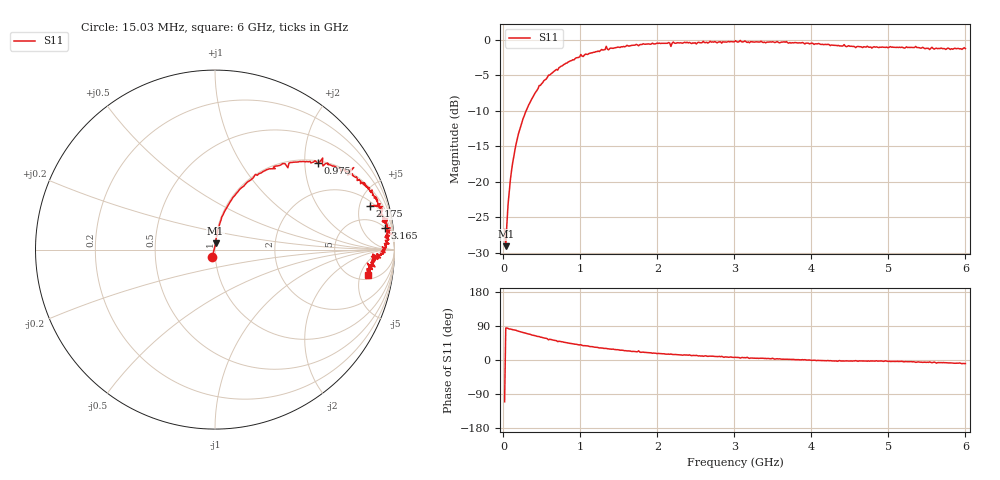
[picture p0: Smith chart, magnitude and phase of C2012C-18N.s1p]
!	Network	Analyzer	HP8753E.07.74:	Oct	30	2002	Serial	No.	JP38451487
!	Hewlett-Packard
!	7	Sep	2009	10:46:32
!	Frequency	S11
#	HZ	S	RI	R	50
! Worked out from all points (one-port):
!   400 points, 15.03 MHz to 6 GHz, reference 50 ohm
!   lowest |S11| = -29.1 dB at 30.03 MHz (marker M1), VSWR 1.07, Z = 50.2 + j3.51 ohm
!   |S11| at or under -10 dB: start of sweep to 295.5 MHz
!   S11 on the Smith chart (normalised r, x): 15.03 MHz: 0.97, -0.08; 975 MHz: 1.06, +2.33; 2.175 GHz: 2.52, +6.25; 3.165 GHz: 5, +14; 6 GHz: 6.09, -6.85
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1.502992e7  -0.0159 -0.0431
3.002985e7  0.00348 0.0349
6.00297e7  0.00803 0.0687
1.050295e8  0.0191 0.118
1.650292e8  0.0376 0.181
2.550287e8  0.0838 0.265
4.650277e8  0.225 0.419
7.650262e8  0.437 0.487
9.750251e8  0.574 0.482
1.335023e9  0.773 0.457
1.365023e9  0.739 0.416
1.515022e9  0.792 0.385
1.725021e9  0.86 0.345
1.755021e9  0.826 0.373
1.785021e9  0.869 0.318
1.93502e9  0.9 0.289
2.145019e9  0.92 0.256
2.175019e9  0.863 0.243
2.205019e9  0.932 0.239
2.265019e9  0.924 0.231
3.015015e9  0.976 0.121
3.075015e9  0.984 0.0847
3.165014e9  0.948 0.121
3.195014e9  0.949 0.0703
3.765011e9  0.949 0.0288
4.515007e9  0.899 -0.0397
5.265004e9  0.881 -0.0687
6e9  0.854 -0.141
